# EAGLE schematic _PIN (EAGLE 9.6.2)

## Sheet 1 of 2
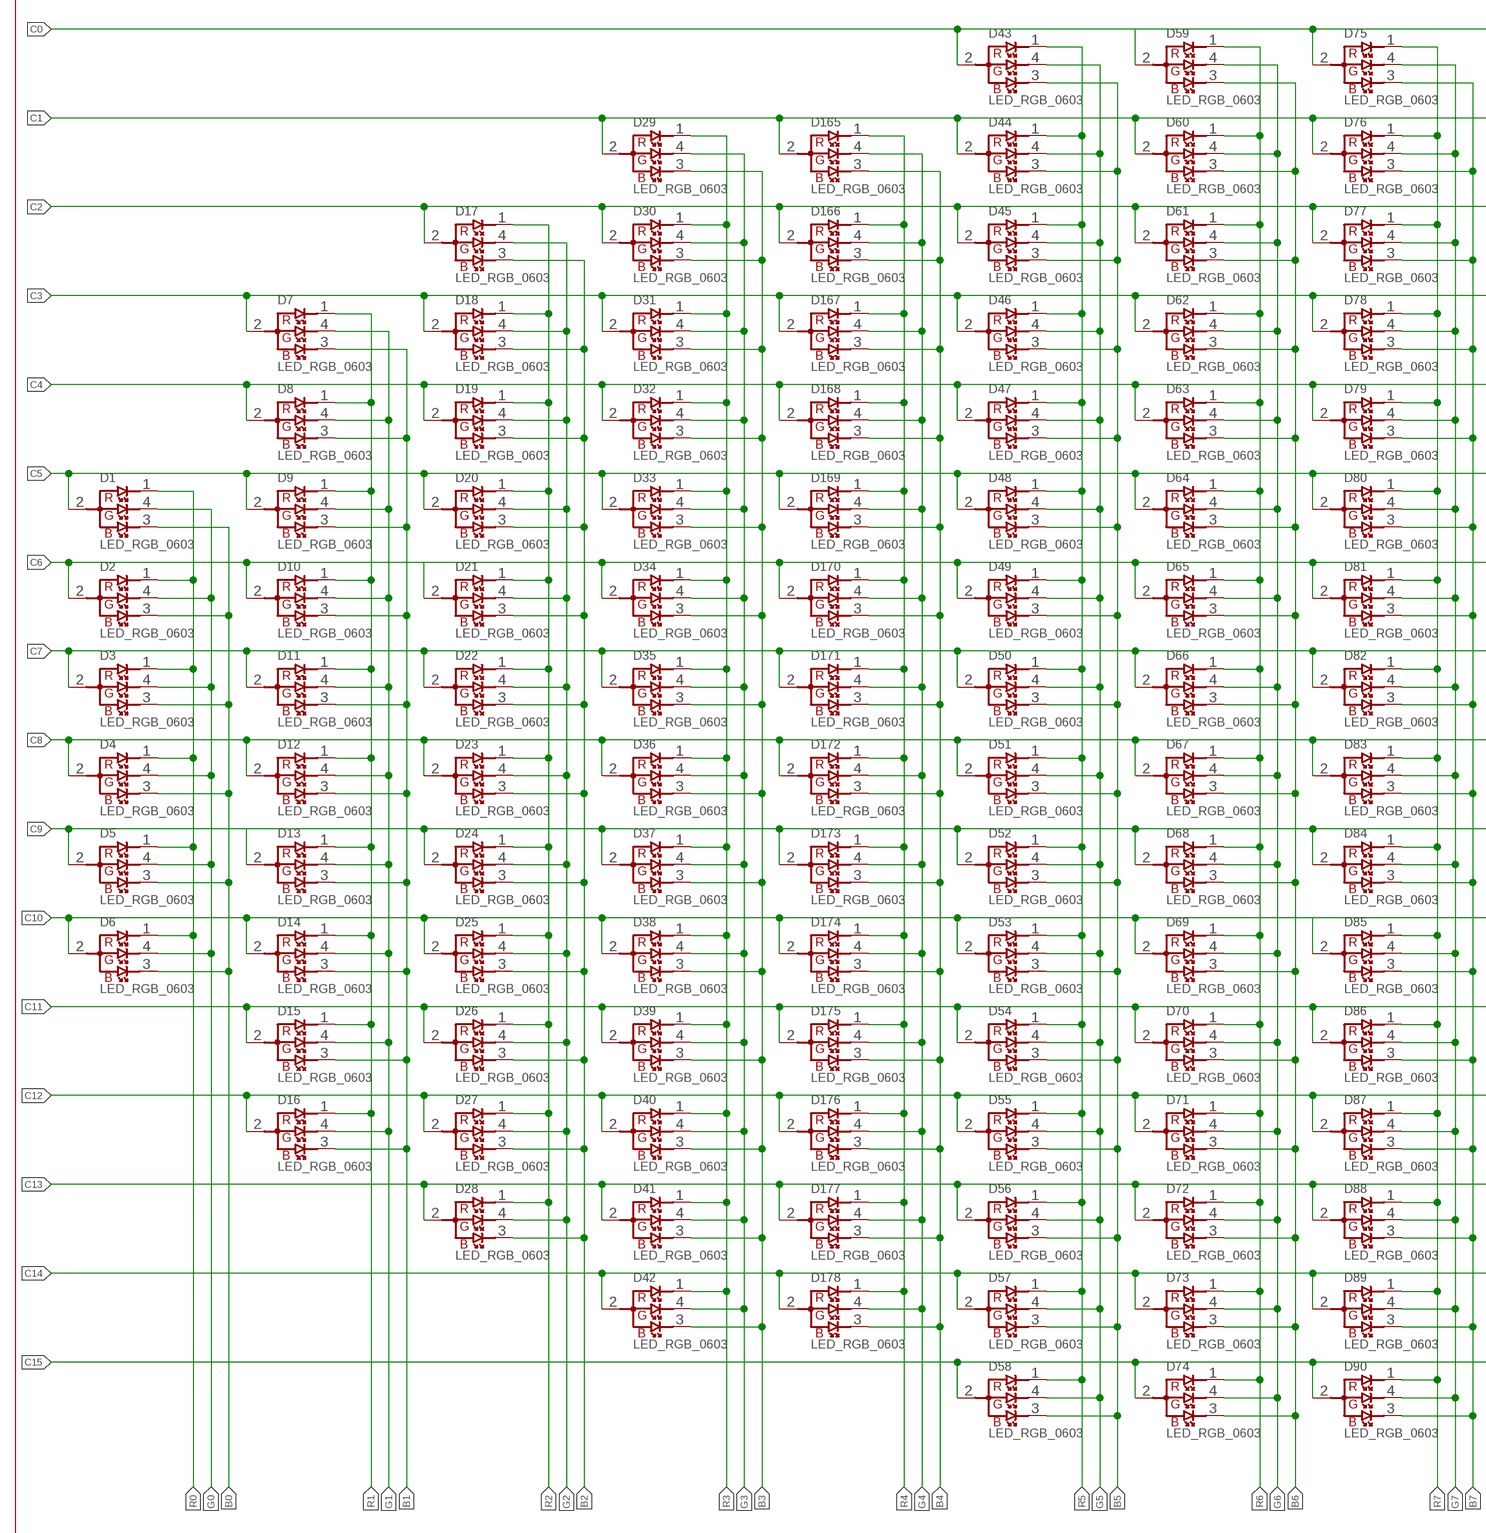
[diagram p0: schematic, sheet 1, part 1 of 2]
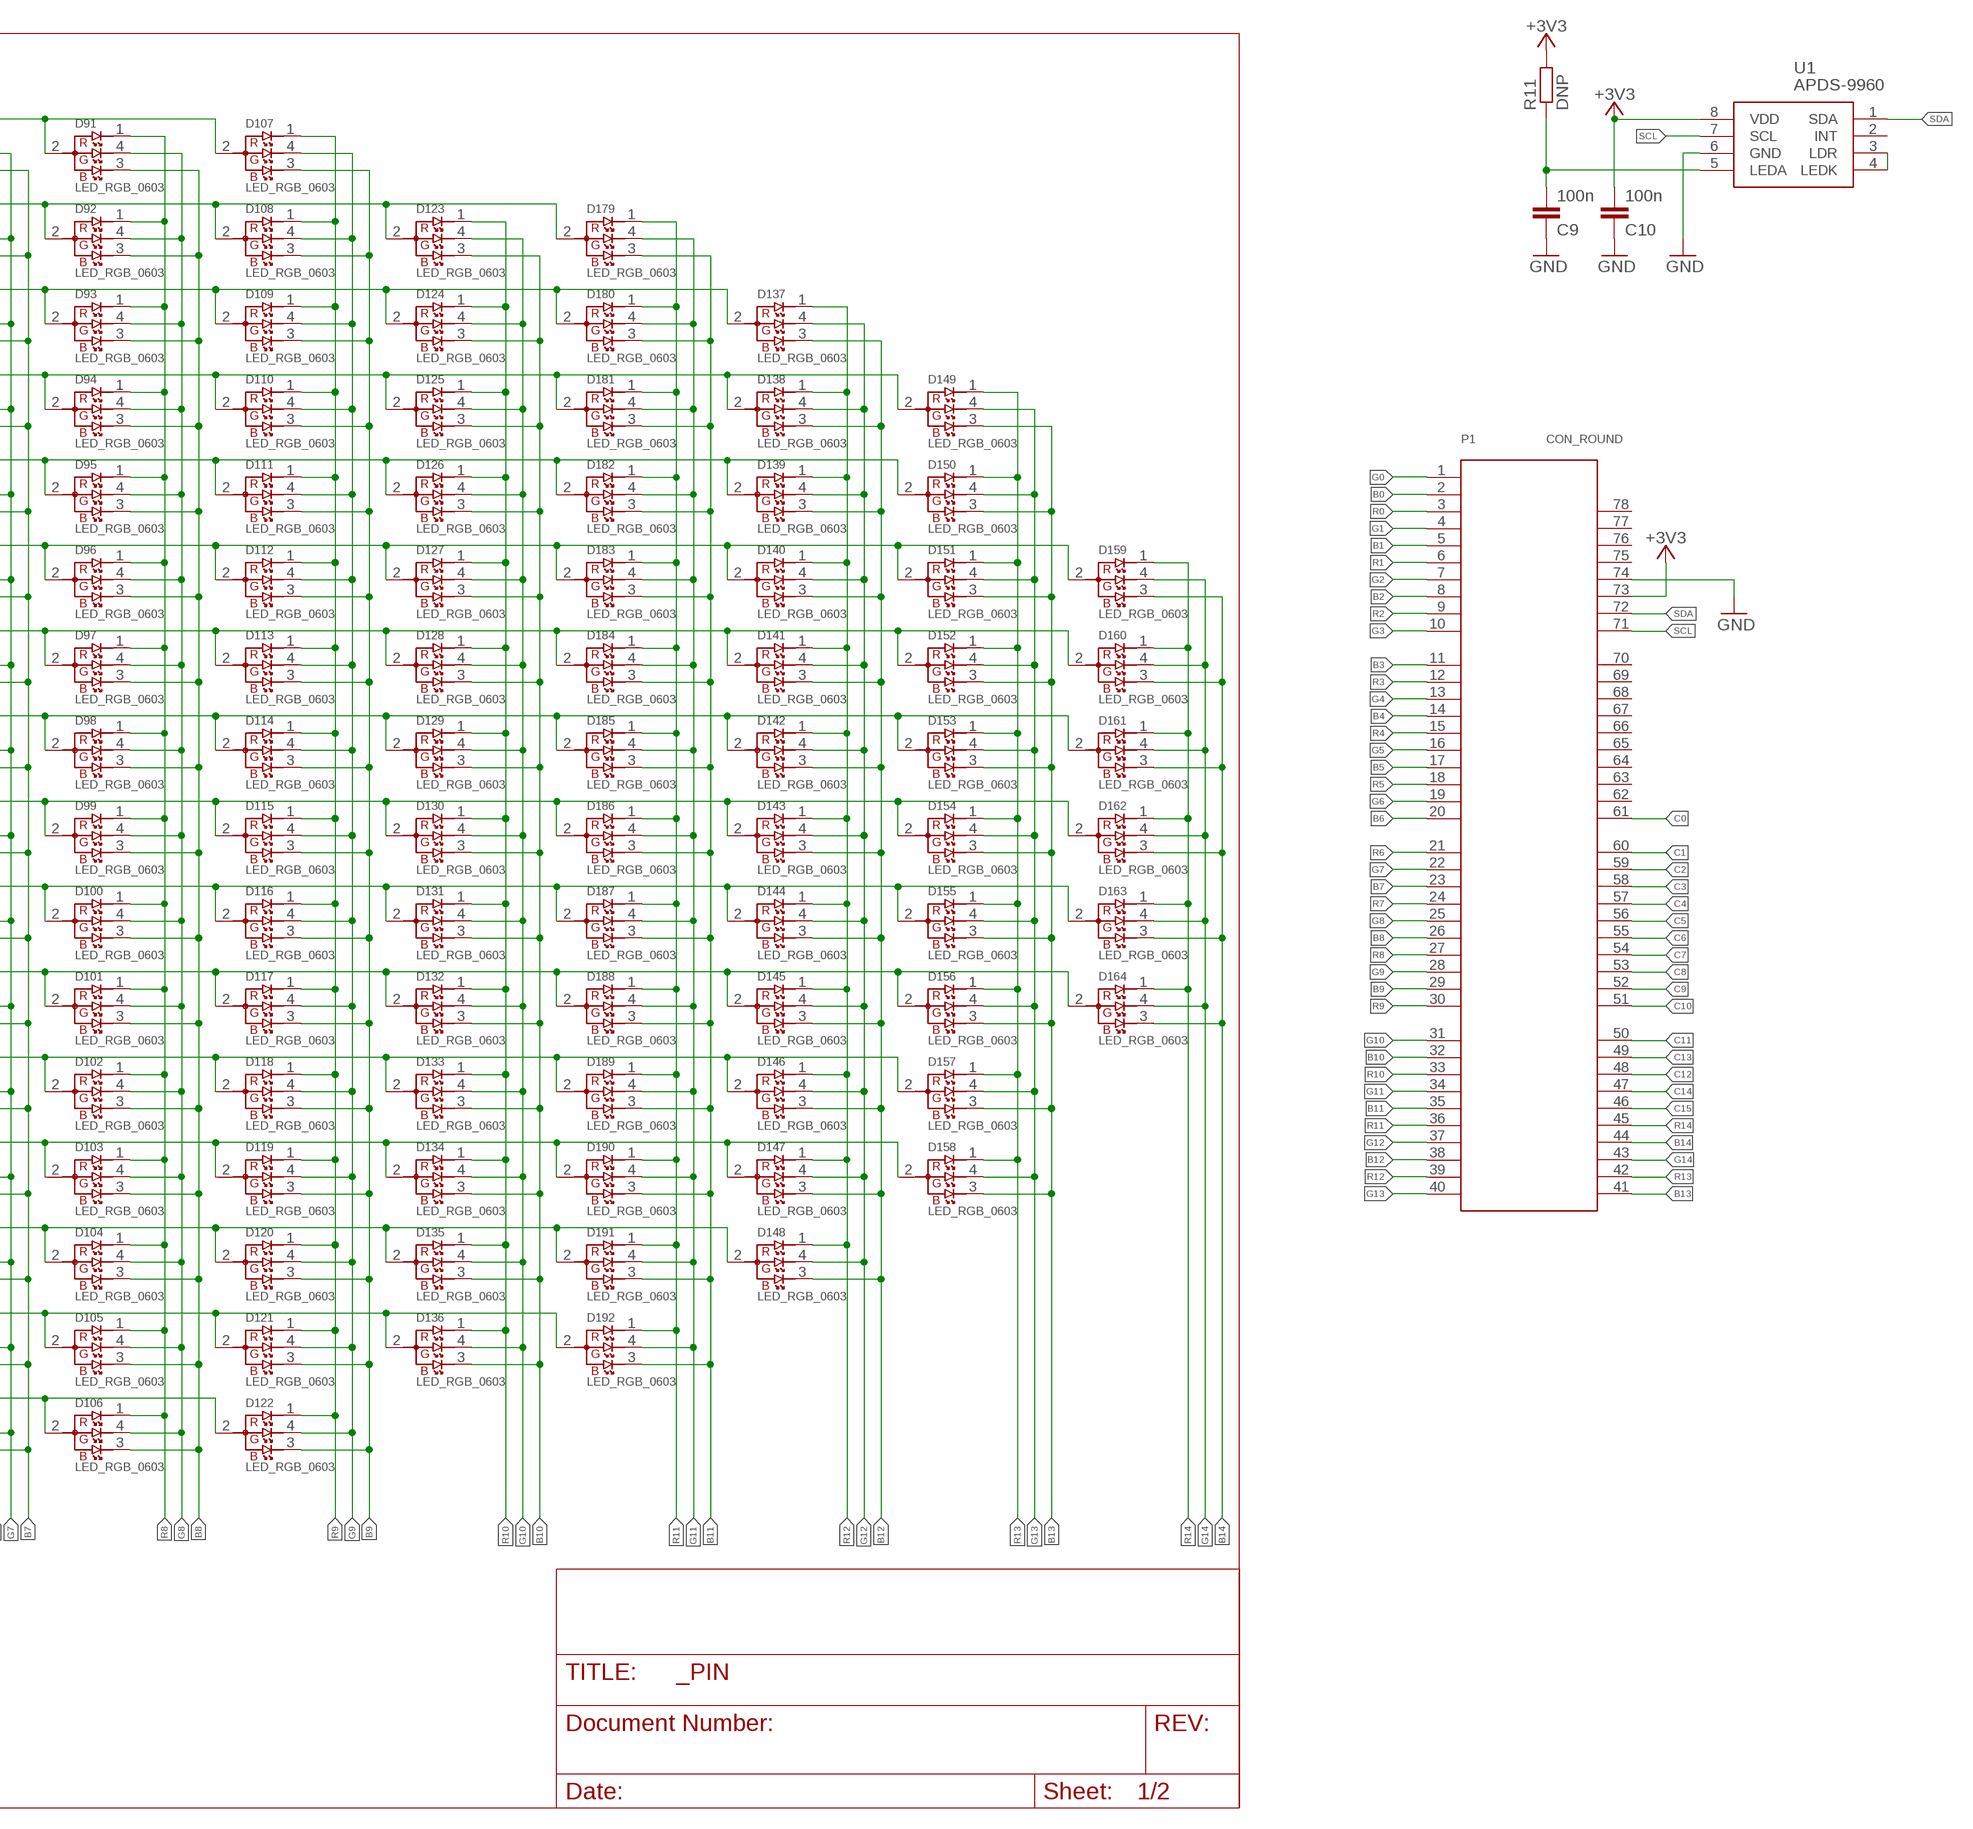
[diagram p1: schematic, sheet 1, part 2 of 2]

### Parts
C9  100n  C-EUC0402K  [C0402K]
C10  100n  C-EUC0402K  [C0402K]
D1  LED_RGB_0603  [LED_RGB_0603]
D2  LED_RGB_0603  [LED_RGB_0603]
D3  LED_RGB_0603  [LED_RGB_0603]
D4  LED_RGB_0603  [LED_RGB_0603]
D5  LED_RGB_0603  [LED_RGB_0603]
D6  LED_RGB_0603  [LED_RGB_0603]
D7  LED_RGB_0603  [LED_RGB_0603]
D8  LED_RGB_0603  [LED_RGB_0603]
D9  LED_RGB_0603  [LED_RGB_0603]
D10  LED_RGB_0603  [LED_RGB_0603]
D11  LED_RGB_0603  [LED_RGB_0603]
D12  LED_RGB_0603  [LED_RGB_0603]
D13  LED_RGB_0603  [LED_RGB_0603]
D14  LED_RGB_0603  [LED_RGB_0603]
D15  LED_RGB_0603  [LED_RGB_0603]
D16  LED_RGB_0603  [LED_RGB_0603]
D17  LED_RGB_0603  [LED_RGB_0603]
D18  LED_RGB_0603  [LED_RGB_0603]
D19  LED_RGB_0603  [LED_RGB_0603]
D20  LED_RGB_0603  [LED_RGB_0603]
D21  LED_RGB_0603  [LED_RGB_0603]
D22  LED_RGB_0603  [LED_RGB_0603]
D23  LED_RGB_0603  [LED_RGB_0603]
D24  LED_RGB_0603  [LED_RGB_0603]
D25  LED_RGB_0603  [LED_RGB_0603]
D26  LED_RGB_0603  [LED_RGB_0603]
D27  LED_RGB_0603  [LED_RGB_0603]
D28  LED_RGB_0603  [LED_RGB_0603]
D29  LED_RGB_0603  [LED_RGB_0603]
D30  LED_RGB_0603  [LED_RGB_0603]
D31  LED_RGB_0603  [LED_RGB_0603]
D32  LED_RGB_0603  [LED_RGB_0603]
D33  LED_RGB_0603  [LED_RGB_0603]
D34  LED_RGB_0603  [LED_RGB_0603]
D35  LED_RGB_0603  [LED_RGB_0603]
D36  LED_RGB_0603  [LED_RGB_0603]
D37  LED_RGB_0603  [LED_RGB_0603]
D38  LED_RGB_0603  [LED_RGB_0603]
D39  LED_RGB_0603  [LED_RGB_0603]
D40  LED_RGB_0603  [LED_RGB_0603]
D41  LED_RGB_0603  [LED_RGB_0603]
D42  LED_RGB_0603  [LED_RGB_0603]
D43  LED_RGB_0603  [LED_RGB_0603]
D44  LED_RGB_0603  [LED_RGB_0603]
D45  LED_RGB_0603  [LED_RGB_0603]
D46  LED_RGB_0603  [LED_RGB_0603]
D47  LED_RGB_0603  [LED_RGB_0603]
D48  LED_RGB_0603  [LED_RGB_0603]
D49  LED_RGB_0603  [LED_RGB_0603]
D50  LED_RGB_0603  [LED_RGB_0603]
D51  LED_RGB_0603  [LED_RGB_0603]
D52  LED_RGB_0603  [LED_RGB_0603]
D53  LED_RGB_0603  [LED_RGB_0603]
D54  LED_RGB_0603  [LED_RGB_0603]
D55  LED_RGB_0603  [LED_RGB_0603]
D56  LED_RGB_0603  [LED_RGB_0603]
D57  LED_RGB_0603  [LED_RGB_0603]
D58  LED_RGB_0603  [LED_RGB_0603]
D59  LED_RGB_0603  [LED_RGB_0603]
D60  LED_RGB_0603  [LED_RGB_0603]
D61  LED_RGB_0603  [LED_RGB_0603]
D62  LED_RGB_0603  [LED_RGB_0603]
D63  LED_RGB_0603  [LED_RGB_0603]
D64  LED_RGB_0603  [LED_RGB_0603]
D65  LED_RGB_0603  [LED_RGB_0603]
D66  LED_RGB_0603  [LED_RGB_0603]
D67  LED_RGB_0603  [LED_RGB_0603]
D68  LED_RGB_0603  [LED_RGB_0603]
D69  LED_RGB_0603  [LED_RGB_0603]
D70  LED_RGB_0603  [LED_RGB_0603]
D71  LED_RGB_0603  [LED_RGB_0603]
D72  LED_RGB_0603  [LED_RGB_0603]
D73  LED_RGB_0603  [LED_RGB_0603]
D74  LED_RGB_0603  [LED_RGB_0603]
D75  LED_RGB_0603  [LED_RGB_0603]
D76  LED_RGB_0603  [LED_RGB_0603]
D77  LED_RGB_0603  [LED_RGB_0603]
D78  LED_RGB_0603  [LED_RGB_0603]
D79  LED_RGB_0603  [LED_RGB_0603]
D80  LED_RGB_0603  [LED_RGB_0603]
D81  LED_RGB_0603  [LED_RGB_0603]
D82  LED_RGB_0603  [LED_RGB_0603]
D83  LED_RGB_0603  [LED_RGB_0603]
D84  LED_RGB_0603  [LED_RGB_0603]
D85  LED_RGB_0603  [LED_RGB_0603]
D86  LED_RGB_0603  [LED_RGB_0603]
D87  LED_RGB_0603  [LED_RGB_0603]
D88  LED_RGB_0603  [LED_RGB_0603]
D89  LED_RGB_0603  [LED_RGB_0603]
D90  LED_RGB_0603  [LED_RGB_0603]
D91  LED_RGB_0603  [LED_RGB_0603]
D92  LED_RGB_0603  [LED_RGB_0603]
D93  LED_RGB_0603  [LED_RGB_0603]
D94  LED_RGB_0603  [LED_RGB_0603]
D95  LED_RGB_0603  [LED_RGB_0603]
D96  LED_RGB_0603  [LED_RGB_0603]
D97  LED_RGB_0603  [LED_RGB_0603]
D98  LED_RGB_0603  [LED_RGB_0603]
D99  LED_RGB_0603  [LED_RGB_0603]
D100  LED_RGB_0603  [LED_RGB_0603]
D101  LED_RGB_0603  [LED_RGB_0603]
D102  LED_RGB_0603  [LED_RGB_0603]
D103  LED_RGB_0603  [LED_RGB_0603]
D104  LED_RGB_0603  [LED_RGB_0603]
D105  LED_RGB_0603  [LED_RGB_0603]
D106  LED_RGB_0603  [LED_RGB_0603]
D107  LED_RGB_0603  [LED_RGB_0603]
D108  LED_RGB_0603  [LED_RGB_0603]
D109  LED_RGB_0603  [LED_RGB_0603]
D110  LED_RGB_0603  [LED_RGB_0603]
D111  LED_RGB_0603  [LED_RGB_0603]
D112  LED_RGB_0603  [LED_RGB_0603]
D113  LED_RGB_0603  [LED_RGB_0603]
D114  LED_RGB_0603  [LED_RGB_0603]
D115  LED_RGB_0603  [LED_RGB_0603]
D116  LED_RGB_0603  [LED_RGB_0603]
D117  LED_RGB_0603  [LED_RGB_0603]
D118  LED_RGB_0603  [LED_RGB_0603]
D119  LED_RGB_0603  [LED_RGB_0603]
D120  LED_RGB_0603  [LED_RGB_0603]
D121  LED_RGB_0603  [LED_RGB_0603]
D122  LED_RGB_0603  [LED_RGB_0603]
D123  LED_RGB_0603  [LED_RGB_0603]
D124  LED_RGB_0603  [LED_RGB_0603]
D125  LED_RGB_0603  [LED_RGB_0603]
D126  LED_RGB_0603  [LED_RGB_0603]
D127  LED_RGB_0603  [LED_RGB_0603]
D128  LED_RGB_0603  [LED_RGB_0603]
D129  LED_RGB_0603  [LED_RGB_0603]
D130  LED_RGB_0603  [LED_RGB_0603]
D131  LED_RGB_0603  [LED_RGB_0603]
D132  LED_RGB_0603  [LED_RGB_0603]
D133  LED_RGB_0603  [LED_RGB_0603]
D134  LED_RGB_0603  [LED_RGB_0603]
D135  LED_RGB_0603  [LED_RGB_0603]
D136  LED_RGB_0603  [LED_RGB_0603]
D137  LED_RGB_0603  [LED_RGB_0603]
D138  LED_RGB_0603  [LED_RGB_0603]
D139  LED_RGB_0603  [LED_RGB_0603]
D140  LED_RGB_0603  [LED_RGB_0603]
D141  LED_RGB_0603  [LED_RGB_0603]
D142  LED_RGB_0603  [LED_RGB_0603]
D143  LED_RGB_0603  [LED_RGB_0603]
D144  LED_RGB_0603  [LED_RGB_0603]
D145  LED_RGB_0603  [LED_RGB_0603]
D146  LED_RGB_0603  [LED_RGB_0603]
D147  LED_RGB_0603  [LED_RGB_0603]
D148  LED_RGB_0603  [LED_RGB_0603]
D149  LED_RGB_0603  [LED_RGB_0603]
D150  LED_RGB_0603  [LED_RGB_0603]
D151  LED_RGB_0603  [LED_RGB_0603]
D152  LED_RGB_0603  [LED_RGB_0603]
D153  LED_RGB_0603  [LED_RGB_0603]
D154  LED_RGB_0603  [LED_RGB_0603]
D155  LED_RGB_0603  [LED_RGB_0603]
D156  LED_RGB_0603  [LED_RGB_0603]
D157  LED_RGB_0603  [LED_RGB_0603]
D158  LED_RGB_0603  [LED_RGB_0603]
D159  LED_RGB_0603  [LED_RGB_0603]
D160  LED_RGB_0603  [LED_RGB_0603]
D161  LED_RGB_0603  [LED_RGB_0603]
D162  LED_RGB_0603  [LED_RGB_0603]
D163  LED_RGB_0603  [LED_RGB_0603]
D164  LED_RGB_0603  [LED_RGB_0603]
D165  LED_RGB_0603  [LED_RGB_0603]
D166  LED_RGB_0603  [LED_RGB_0603]
D167  LED_RGB_0603  [LED_RGB_0603]
D168  LED_RGB_0603  [LED_RGB_0603]
D169  LED_RGB_0603  [LED_RGB_0603]
D170  LED_RGB_0603  [LED_RGB_0603]
D171  LED_RGB_0603  [LED_RGB_0603]
D172  LED_RGB_0603  [LED_RGB_0603]
D173  LED_RGB_0603  [LED_RGB_0603]
D174  LED_RGB_0603  [LED_RGB_0603]
D175  LED_RGB_0603  [LED_RGB_0603]
D176  LED_RGB_0603  [LED_RGB_0603]
D177  LED_RGB_0603  [LED_RGB_0603]
D178  LED_RGB_0603  [LED_RGB_0603]
D179  LED_RGB_0603  [LED_RGB_0603]
D180  LED_RGB_0603  [LED_RGB_0603]
D181  LED_RGB_0603  [LED_RGB_0603]
D182  LED_RGB_0603  [LED_RGB_0603]
D183  LED_RGB_0603  [LED_RGB_0603]
D184  LED_RGB_0603  [LED_RGB_0603]
D185  LED_RGB_0603  [LED_RGB_0603]
D186  LED_RGB_0603  [LED_RGB_0603]
D187  LED_RGB_0603  [LED_RGB_0603]
D188  LED_RGB_0603  [LED_RGB_0603]
D189  LED_RGB_0603  [LED_RGB_0603]
D190  LED_RGB_0603  [LED_RGB_0603]
D191  LED_RGB_0603  [LED_RGB_0603]
D192  LED_RGB_0603  [LED_RGB_0603]
P1  CON_ROUND  [CONNECTOR_61]
R11  DNP  R-EU_R0402  [R0402]
U1  APDS-9960  [APDS-9950]

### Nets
+3V3: C10.2 P1.73 R11.2 U1.8(VDD)
B0: D1.3(B) D2.3(B) D3.3(B) D4.3(B) D5.3(B) D6.3(B) P1.2
B1: D7.3(B) D8.3(B) D9.3(B) D10.3(B) D11.3(B) D12.3(B) D13.3(B) D14.3(B) D15.3(B) D16.3(B) P1.5
B2: D17.3(B) D18.3(B) D19.3(B) D20.3(B) D21.3(B) D22.3(B) D23.3(B) D24.3(B) D25.3(B) D26.3(B) D27.3(B) D28.3(B) P1.8
B3: D29.3(B) D30.3(B) D31.3(B) D32.3(B) D33.3(B) D34.3(B) D35.3(B) D36.3(B) D37.3(B) D38.3(B) D39.3(B) D40.3(B) D41.3(B) D42.3(B) P1.11
B4: D165.3(B) D166.3(B) D167.3(B) D168.3(B) D169.3(B) D170.3(B) D171.3(B) D172.3(B) D173.3(B) D174.3(B) D175.3(B) D176.3(B) D177.3(B) D178.3(B) P1.14
B5: D43.3(B) D44.3(B) D45.3(B) D46.3(B) D47.3(B) D48.3(B) D49.3(B) D50.3(B) D51.3(B) D52.3(B) D53.3(B) D54.3(B) D55.3(B) D56.3(B) D57.3(B) D58.3(B) P1.17
B6: D59.3(B) D60.3(B) D61.3(B) D62.3(B) D63.3(B) D64.3(B) D65.3(B) D66.3(B) D67.3(B) D68.3(B) D69.3(B) D70.3(B) D71.3(B) D72.3(B) D73.3(B) D74.3(B) P1.20
B7: D75.3(B) D76.3(B) D77.3(B) D78.3(B) D79.3(B) D80.3(B) D81.3(B) D82.3(B) D83.3(B) D84.3(B) D85.3(B) D86.3(B) D87.3(B) D88.3(B) D89.3(B) D90.3(B) P1.23
B8: D91.3(B) D92.3(B) D93.3(B) D94.3(B) D95.3(B) D96.3(B) D97.3(B) D98.3(B) D99.3(B) D100.3(B) D101.3(B) D102.3(B) D103.3(B) D104.3(B) D105.3(B) D106.3(B) P1.26
B9: D107.3(B) D108.3(B) D109.3(B) D110.3(B) D111.3(B) D112.3(B) D113.3(B) D114.3(B) D115.3(B) D116.3(B) D117.3(B) D118.3(B) D119.3(B) D120.3(B) D121.3(B) D122.3(B) P1.29
B10: D123.3(B) D124.3(B) D125.3(B) D126.3(B) D127.3(B) D128.3(B) D129.3(B) D130.3(B) D131.3(B) D132.3(B) D133.3(B) D134.3(B) D135.3(B) D136.3(B) P1.32
B11: D179.3(B) D180.3(B) D181.3(B) D182.3(B) D183.3(B) D184.3(B) D185.3(B) D186.3(B) D187.3(B) D188.3(B) D189.3(B) D190.3(B) D191.3(B) D192.3(B) P1.35
B12: D137.3(B) D138.3(B) D139.3(B) D140.3(B) D141.3(B) D142.3(B) D143.3(B) D144.3(B) D145.3(B) D146.3(B) D147.3(B) D148.3(B) P1.38
B13: D149.3(B) D150.3(B) D151.3(B) D152.3(B) D153.3(B) D154.3(B) D155.3(B) D156.3(B) D157.3(B) D158.3(B) P1.41
B14: D159.3(B) D160.3(B) D161.3(B) D162.3(B) D163.3(B) D164.3(B) P1.44
C0: D43.2(CA) D59.2(CA) D75.2(CA) D91.2(CA) D107.2(CA) P1.61
C1: D29.2(CA) D44.2(CA) D60.2(CA) D76.2(CA) D92.2(CA) D108.2(CA) D123.2(CA) D165.2(CA) D179.2(CA) P1.60
C2: D17.2(CA) D30.2(CA) D45.2(CA) D61.2(CA) D77.2(CA) D93.2(CA) D109.2(CA) D124.2(CA) D137.2(CA) D166.2(CA) D180.2(CA) P1.59
C3: D7.2(CA) D18.2(CA) D31.2(CA) D46.2(CA) D62.2(CA) D78.2(CA) D94.2(CA) D110.2(CA) D125.2(CA) D138.2(CA) D149.2(CA) D167.2(CA) D181.2(CA) P1.58
C4: D8.2(CA) D19.2(CA) D32.2(CA) D47.2(CA) D63.2(CA) D79.2(CA) D95.2(CA) D111.2(CA) D126.2(CA) D139.2(CA) D150.2(CA) D168.2(CA) D182.2(CA) P1.57
C5: D1.2(CA) D9.2(CA) D20.2(CA) D33.2(CA) D48.2(CA) D64.2(CA) D80.2(CA) D96.2(CA) D112.2(CA) D127.2(CA) D140.2(CA) D151.2(CA) D159.2(CA) D169.2(CA) D183.2(CA) P1.56
C6: D2.2(CA) D10.2(CA) D21.2(CA) D34.2(CA) D49.2(CA) D65.2(CA) D81.2(CA) D97.2(CA) D113.2(CA) D128.2(CA) D141.2(CA) D152.2(CA) D160.2(CA) D170.2(CA) D184.2(CA) P1.55
C7: D3.2(CA) D11.2(CA) D22.2(CA) D35.2(CA) D50.2(CA) D66.2(CA) D82.2(CA) D98.2(CA) D114.2(CA) D129.2(CA) D142.2(CA) D153.2(CA) D161.2(CA) D171.2(CA) D185.2(CA) P1.54
C8: D4.2(CA) D12.2(CA) D23.2(CA) D36.2(CA) D51.2(CA) D67.2(CA) D83.2(CA) D99.2(CA) D115.2(CA) D130.2(CA) D143.2(CA) D154.2(CA) D162.2(CA) D172.2(CA) D186.2(CA) P1.53
C9: D5.2(CA) D13.2(CA) D24.2(CA) D37.2(CA) D52.2(CA) D68.2(CA) D84.2(CA) D100.2(CA) D116.2(CA) D131.2(CA) D144.2(CA) D155.2(CA) D163.2(CA) D173.2(CA) D187.2(CA) P1.52
C10: D6.2(CA) D14.2(CA) D25.2(CA) D38.2(CA) D53.2(CA) D69.2(CA) D85.2(CA) D101.2(CA) D117.2(CA) D132.2(CA) D145.2(CA) D156.2(CA) D164.2(CA) D174.2(CA) D188.2(CA) P1.51
C11: D15.2(CA) D26.2(CA) D39.2(CA) D54.2(CA) D70.2(CA) D86.2(CA) D102.2(CA) D118.2(CA) D133.2(CA) D146.2(CA) D157.2(CA) D175.2(CA) D189.2(CA) P1.50
C12: D16.2(CA) D27.2(CA) D40.2(CA) D55.2(CA) D71.2(CA) D87.2(CA) D103.2(CA) D119.2(CA) D134.2(CA) D147.2(CA) D158.2(CA) D176.2(CA) D190.2(CA) P1.48
C13: D28.2(CA) D41.2(CA) D56.2(CA) D72.2(CA) D88.2(CA) D104.2(CA) D120.2(CA) D135.2(CA) D148.2(CA) D177.2(CA) D191.2(CA) P1.49
C14: D42.2(CA) D57.2(CA) D73.2(CA) D89.2(CA) D105.2(CA) D121.2(CA) D136.2(CA) D178.2(CA) D192.2(CA) P1.47
C15: D58.2(CA) D74.2(CA) D90.2(CA) D106.2(CA) D122.2(CA) P1.46
G0: D1.4(G) D2.4(G) D3.4(G) D4.4(G) D5.4(G) D6.4(G) P1.1
G1: D7.4(G) D8.4(G) D9.4(G) D10.4(G) D11.4(G) D12.4(G) D13.4(G) D14.4(G) D15.4(G) D16.4(G) P1.4
G2: D17.4(G) D18.4(G) D19.4(G) D20.4(G) D21.4(G) D22.4(G) D23.4(G) D24.4(G) D25.4(G) D26.4(G) D27.4(G) D28.4(G) P1.7
G3: D29.4(G) D30.4(G) D31.4(G) D32.4(G) D33.4(G) D34.4(G) D35.4(G) D36.4(G) D37.4(G) D38.4(G) D39.4(G) D40.4(G) D41.4(G) D42.4(G) P1.10
G4: D165.4(G) D166.4(G) D167.4(G) D168.4(G) D169.4(G) D170.4(G) D171.4(G) D172.4(G) D173.4(G) D174.4(G) D175.4(G) D176.4(G) D177.4(G) D178.4(G) P1.13
G5: D43.4(G) D44.4(G) D45.4(G) D46.4(G) D47.4(G) D48.4(G) D49.4(G) D50.4(G) D51.4(G) D52.4(G) D53.4(G) D54.4(G) D55.4(G) D56.4(G) D57.4(G) D58.4(G) P1.16
G6: D59.4(G) D60.4(G) D61.4(G) D62.4(G) D63.4(G) D64.4(G) D65.4(G) D66.4(G) D67.4(G) D68.4(G) D69.4(G) D70.4(G) D71.4(G) D72.4(G) D73.4(G) D74.4(G) P1.19
G7: D75.4(G) D76.4(G) D77.4(G) D78.4(G) D79.4(G) D80.4(G) D81.4(G) D82.4(G) D83.4(G) D84.4(G) D85.4(G) D86.4(G) D87.4(G) D88.4(G) D89.4(G) D90.4(G) P1.22
G8: D91.4(G) D92.4(G) D93.4(G) D94.4(G) D95.4(G) D96.4(G) D97.4(G) D98.4(G) D99.4(G) D100.4(G) D101.4(G) D102.4(G) D103.4(G) D104.4(G) D105.4(G) D106.4(G) P1.25
G9: D107.4(G) D108.4(G) D109.4(G) D110.4(G) D111.4(G) D112.4(G) D113.4(G) D114.4(G) D115.4(G) D116.4(G) D117.4(G) D118.4(G) D119.4(G) D120.4(G) D121.4(G) D122.4(G) P1.28
G10: D123.4(G) D124.4(G) D125.4(G) D126.4(G) D127.4(G) D128.4(G) D129.4(G) D130.4(G) D131.4(G) D132.4(G) D133.4(G) D134.4(G) D135.4(G) D136.4(G) P1.31
G11: D179.4(G) D180.4(G) D181.4(G) D182.4(G) D183.4(G) D184.4(G) D185.4(G) D186.4(G) D187.4(G) D188.4(G) D189.4(G) D190.4(G) D191.4(G) D192.4(G) P1.34
G12: D137.4(G) D138.4(G) D139.4(G) D140.4(G) D141.4(G) D142.4(G) D143.4(G) D144.4(G) D145.4(G) D146.4(G) D147.4(G) D148.4(G) P1.37
G13: D149.4(G) D150.4(G) D151.4(G) D152.4(G) D153.4(G) D154.4(G) D155.4(G) D156.4(G) D157.4(G) D158.4(G) P1.40
G14: D159.4(G) D160.4(G) D161.4(G) D162.4(G) D163.4(G) D164.4(G) P1.43
GND: C9.1 C10.1 P1.74 U1.6(GND)
N$38: U1.3(LDR) U1.4(LEDK)
N$40: C9.2 R11.1 U1.5(LEDA)
R0: D1.1(R) D2.1(R) D3.1(R) D4.1(R) D5.1(R) D6.1(R) P1.3
R1: D7.1(R) D8.1(R) D9.1(R) D10.1(R) D11.1(R) D12.1(R) D13.1(R) D14.1(R) D15.1(R) D16.1(R) P1.6
R2: D17.1(R) D18.1(R) D19.1(R) D20.1(R) D21.1(R) D22.1(R) D23.1(R) D24.1(R) D25.1(R) D26.1(R) D27.1(R) D28.1(R) P1.9
R3: D29.1(R) D30.1(R) D31.1(R) D32.1(R) D33.1(R) D34.1(R) D35.1(R) D36.1(R) D37.1(R) D38.1(R) D39.1(R) D40.1(R) D41.1(R) D42.1(R) P1.12
R4: D165.1(R) D166.1(R) D167.1(R) D168.1(R) D169.1(R) D170.1(R) D171.1(R) D172.1(R) D173.1(R) D174.1(R) D175.1(R) D176.1(R) D177.1(R) D178.1(R) P1.15
R5: D43.1(R) D44.1(R) D45.1(R) D46.1(R) D47.1(R) D48.1(R) D49.1(R) D50.1(R) D51.1(R) D52.1(R) D53.1(R) D54.1(R) D55.1(R) D56.1(R) D57.1(R) D58.1(R) P1.18
R6: D59.1(R) D60.1(R) D61.1(R) D62.1(R) D63.1(R) D64.1(R) D65.1(R) D66.1(R) D67.1(R) D68.1(R) D69.1(R) D70.1(R) D71.1(R) D72.1(R) D73.1(R) D74.1(R) P1.21
R7: D75.1(R) D76.1(R) D77.1(R) D78.1(R) D79.1(R) D80.1(R) D81.1(R) D82.1(R) D83.1(R) D84.1(R) D85.1(R) D86.1(R) D87.1(R) D88.1(R) D89.1(R) D90.1(R) P1.24
R8: D91.1(R) D92.1(R) D93.1(R) D94.1(R) D95.1(R) D96.1(R) D97.1(R) D98.1(R) D99.1(R) D100.1(R) D101.1(R) D102.1(R) D103.1(R) D104.1(R) D105.1(R) D106.1(R) P1.27
R9: D107.1(R) D108.1(R) D109.1(R) D110.1(R) D111.1(R) D112.1(R) D113.1(R) D114.1(R) D115.1(R) D116.1(R) D117.1(R) D118.1(R) D119.1(R) D120.1(R) D121.1(R) D122.1(R) P1.30
R10: D123.1(R) D124.1(R) D125.1(R) D126.1(R) D127.1(R) D128.1(R) D129.1(R) D130.1(R) D131.1(R) D132.1(R) D133.1(R) D134.1(R) D135.1(R) D136.1(R) P1.33
R11: D179.1(R) D180.1(R) D181.1(R) D182.1(R) D183.1(R) D184.1(R) D185.1(R) D186.1(R) D187.1(R) D188.1(R) D189.1(R) D190.1(R) D191.1(R) D192.1(R) P1.36
R12: D137.1(R) D138.1(R) D139.1(R) D140.1(R) D141.1(R) D142.1(R) D143.1(R) D144.1(R) D145.1(R) D146.1(R) D147.1(R) D148.1(R) P1.39
R13: D149.1(R) D150.1(R) D151.1(R) D152.1(R) D153.1(R) D154.1(R) D155.1(R) D156.1(R) D157.1(R) D158.1(R) P1.42
R14: D159.1(R) D160.1(R) D161.1(R) D162.1(R) D163.1(R) D164.1(R) P1.45
SCL: P1.71 U1.7(SCL)
SDA: P1.72 U1.1(SDA)
Unconnected: P1.62 P1.63 P1.64 P1.65 P1.66 P1.67 P1.68 P1.69 P1.70 P1.75 P1.76 P1.77 P1.78 U1.2(INT)

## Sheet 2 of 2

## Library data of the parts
C9 C10 = my_rcl:C-EU: CAPACITOR, European symbol; SPICEPREFIX: C
D1-D192 = GUIDO_PCB_LIB:LED_RGB_0603
P1 = GUIDO_PCB_LIB:CON_ROUND
R11 = my_rcl:R-EU_: RESISTOR, European symbol; SPICEPREFIX: R
U1 = APDS-9960:APDS-9960: BROADCOM LIMITED - APDS-9960 - SENSOR, PROXIMITY/GESTURE, 2.4V TO 3.6V Source: Datasheet; ARROW_PART_NUMBER: APDS-9960; DESCRIPTION: BROADCOM LIMITED - APDS-9960 - SENSOR, PROXIMITY/GESTURE, 2.4V TO 3.6V; HEIGHT: mm; MANUFACTURER_NAME: Avago Technologies; MANUFACTURER_PART_NUMBER: APDS-9960; MOUSER_PART_NUMBER: 630-APDS-9960; MOUSER_PRICE-STOCK: https://www.mouser.co.uk/ProductDetail/Broadcom-Avago/APDS-9960?qs=9j6qqDjiC68hPiaH59tKpQ%3D%3D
